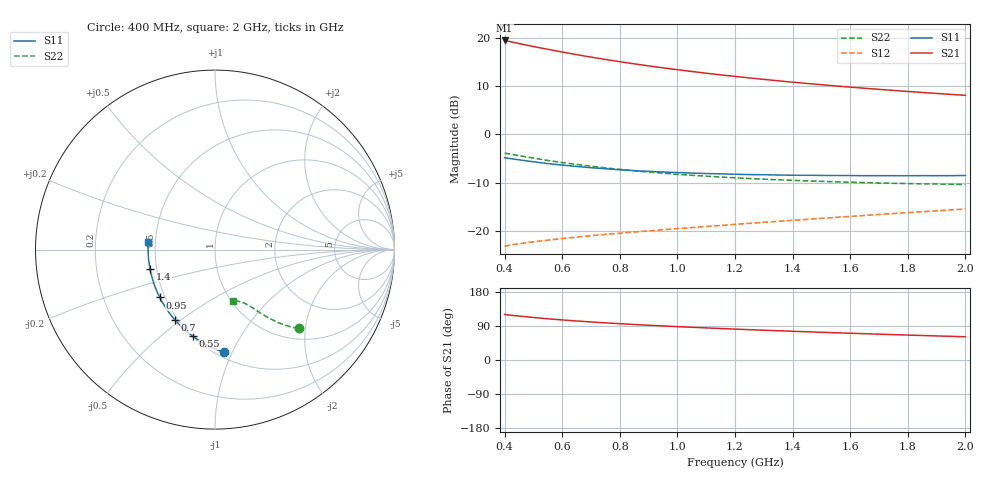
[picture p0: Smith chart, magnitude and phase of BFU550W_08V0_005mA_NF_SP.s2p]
! Filename:  P:\Prog\Test\Noise\ATS_data\Testdata_Net\06 Compressed Noise after Statistics\BFU550W_APM2013_11_D05_08p0V_005mA_NF_CM01_D.sf
! Date/Time: Tue 26/Mar/2013 16:25:24
! BFU550W_APM2013_11_D05_08p0V_1to35mA_NF_CM01_Bias4_R.sf
! Noise Parameter Data File
! BFU550W_APM2013_11_D05_08p0V_1to35mA_NF_CM01
! Date/time: Mon Mar 25 14:39:45 2013
! VAR V_out= 8.000000
! VAR I_out= 4.995000
! VAR V_in= 0.804400
! VAR I_in= 0.049605
! Device data file deembeded for feedlines and parallel
! Original file: \06 Compressed Noise after Statistics\BFU550W_APM2013_11_D05_08p0V_005mA_NF_CM01_R.sf
! Feed-files: PR019V01_070313_Feed1.s2p, PR019V01_070313_Feed2.s2p
! Parallel-file: PR019V01_070313_Par.s2p
# MHz S MA R 50
!  Freq-MHz  S11-mag  S11-arg  S21-mag  S21-arg  S12-mag  S12-arg  S22-mag  S22-arg
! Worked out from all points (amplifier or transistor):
!   37 points, 400 MHz to 2 GHz, reference 50 ohm
!   highest |S21| = 19.5 dB at 400 MHz (marker M1)
!   |S21| within 3 dB of that: start of sweep to 655.2 MHz
!   unconditionally stable (mu >= 1): 1.736 GHz to end of sweep
!   at 500 MHz: K = 0.52, MSG = 20.3 dB, |S12| = -22.3 dB
!   at 1.1 GHz: K = 0.86, MSG = 15.9 dB, |S12| = -19.1 dB
!   at 2 GHz: K = 1.02, MAG = 11.0 dB, |S12| = -15.5 dB
!   lowest NFmin = 0.57 dB at 440 MHz
!   S11 on the Smith chart (normalised r, x): 400 MHz: 0.54, -0.93; 550 MHz: 0.50, -0.64; 700 MHz: 0.48, -0.47; 950 MHz: 0.47, -0.30; 1.4 GHz: 0.46, -0.11; 2 GHz: 0.46, +0.04
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400  0.5737 -85.1  9.481 120.1  0.06902 54.6  0.64 -43.3
420  0.5614 -88.0  9.201 118.4  0.07072 54.0  0.6246 -44.3
440  0.5503 -90.8  8.938 116.7  0.07234 53.4  0.6093 -45.2
480  0.5297 -96.0  8.429 113.7  0.07523 52.6  0.581 -46.8
500  0.52 -98.7  8.198 112.2  0.07658 52.2  0.5676 -47.5
550  0.4976 -104.5  7.676 108.8  0.07975 51.6  0.5368 -49.2
600  0.4807 -110.0  7.193 105.7  0.08288 51.1  0.5101 -50.5
650  0.4649 -114.9  6.753 103.0  0.08582 50.9  0.4881 -51.6
700  0.4512 -119.7  6.369 100.4  0.08862 50.8  0.4674 -52.8
750  0.4403 -124.0  6.016 98.0  0.09138 50.9  0.4495 -53.6
800  0.4293 -128.2  5.703 95.8  0.09413 51.0  0.4339 -54.5
850  0.4207 -132.2  5.418 93.7  0.09682 51.1  0.4193 -55.2
950  0.4069 -139.1  4.925 89.8  0.1022 51.7  0.3956 -56.6
1050  0.3968 -145.5  4.512 86.3  0.1077 52.4  0.3763 -57.9
1150  0.3893 -151.4  4.163 83.1  0.1133 52.9  0.3613 -59.1
1200  0.3857 -153.9  4.011 81.5  0.1162 53.3  0.3546 -59.8
1300  0.3813 -159.0  3.735 78.6  0.1221 53.9  0.3428 -61.0
1400  0.3771 -163.7  3.496 75.8  0.1281 54.5  0.3336 -62.1
1500  0.3751 -168.0  3.288 73.2  0.1343 55.1  0.3258 -63.6
1650  0.3728 -174.2  3.02 69.4  0.144 55.8  0.3161 -65.6
1750  0.3728 -177.7  2.869 67.0  0.1506 56.2  0.3106 -67.0
2000  0.3745 173.8  2.551 61.3  0.1679 56.8  0.302 -71.1
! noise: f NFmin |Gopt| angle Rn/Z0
400  0.5854  0.1807  46.22  0.0964
460  0.5953  0.183  49.48  0.0972
600  0.6151  0.181  62.19  0.1023
800  0.668  0.1951  77.69  0.0923
1000  0.7123  0.2105  92.86  0.09
1200  0.7052  0.2322  108.3  0.088
1400  0.7745  0.2524  127.5  0.0773
1600  0.7538  0.2866  145.4  0.0628
1800  0.8407  0.3116  154.7  0.0593
2000  0.88  0.3389  166.3  0.0538
